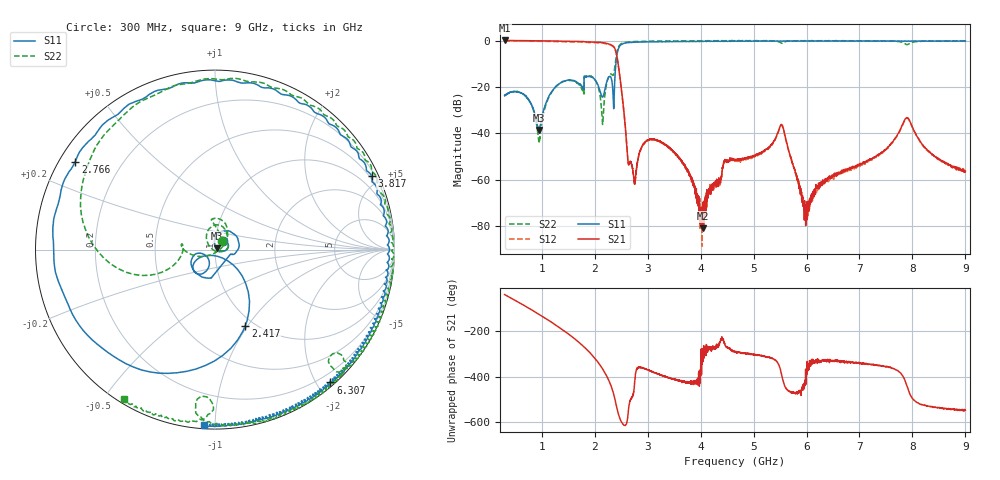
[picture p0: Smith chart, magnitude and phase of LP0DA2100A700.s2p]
!Agilent Technologies,E8358A,US41080443,A.07.50.56
!Agilent E8358A: A.07.50.56
!Date: Friday, August 05, 2016 08:45:06
!Correction: S11(Full 2 Port(1,2))
!S21(Full 2 Port(1,2))
!S12(Full 2 Port(1,2))
!S22(Full 2 Port(1,2))
!S2P File: Measurements: S11, S21, S12, S22:Log Frequency Sweep
# Hz S  dB  R 50
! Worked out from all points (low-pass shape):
!   6401 points, 300 MHz to 9 GHz, reference 50 ohm
!   highest |S21| = 0.06 dB at 301.1 MHz (marker M1); lowest = -81.0 dB at 4.043 GHz (marker M2)
!   |S21| within 3 dB of the highest: start of sweep to 2.371 GHz
!   lowest |S11| = -38.6 dB at 941.5 MHz (marker M3), VSWR 1.02, Z = 51 + j0.676 ohm
!   |S11| at or under -10 dB: start of sweep to 2.401 GHz
!   |S22| runs from -43.7 to 0.0 dB; largest |S21 - S12| = 0.028
!   S11 on the Smith chart (normalised r, x): 300 MHz: 1.09, +0.11; 2.417 GHz: 0.91, -0.98; 2.766 GHz: 0.05, +0.29; 3.817 GHz: 0.38, +4.44; 6.307 GHz: 0.06, -2.19; 9 GHz: 0.02, -0.94
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3e8  -23.71 47.7  0.06 -38.9  -0.17 -38.7  -23.78 50.7
3.011181e8  -23.71 47.7  0.06 -39.0  -0.18 -38.9  -23.74 50.5
7.380687e8  -24.97 -6.4  -0.03 -96.3  -0.25 -96.1  -25.12 -4.8
9.41463e8  -38.57 34.2  -0.05 -124.4  -0.28 -124.3  -42.71 -88.3
1.236527e9  -20.65 77.5  -0.17 -168.1  -0.40 -168.0  -20.78 121.5
1.75044e9  -19.54 -14.4  -0.39 101.6  -0.62 101.8  -20.48 43.3
1.985394e9  -16.36 -151.4  -0.65 46.8  -0.87 47.0  -16.18 67.7
2.137608e9  -24.21 -147.9  -0.84 -0.5  -1.07 -0.3  -32.54 -4.4
2.307614e9  -15.90 -139.8  -1.81 -78.4  -2.04 -78.3  -14.43 171.0
2.416812e9  -6.79 -68.4  -6.30 -173.8  -6.52 -173.8  -5.45 -167.5
2.632702e9  -0.92 178.7  -52.57 162.2  -52.62 161.5  -0.62 107.6
2.766089e9  -0.72 147.8  -60.06 -37.2  -60.10 -36.2  -0.38 84.9
3.201372e9  -0.54 81.2  -43.18 -28.0  -43.38 -28.0  -0.23 39.9
3.817078e9  -0.32 25.2  -58.84 -63.7  -59.23 -65.1  -0.05 3.4
4.042569e9  -0.39 11.3  -81.04 37.4  -77.62 7.1  -0.14 -5.6
4.651453e9  -0.21 -14.2  -51.54 69.1  -51.54 69.1  0.01 -24.3
5.525454e9  -0.22 -36.1  -36.23 -25.8  -36.49 -25.2  -1.12 -44.0
6.102778e9  -0.12 -45.7  -68.85 36.8  -69.21 15.2  -0.01 -52.7
6.307208e9  -0.17 -49.0  -60.12 34.1  -61.97 30.3  -0.06 -56.8
7.552286e9  -0.23 -69.5  -45.69 2.6  -45.83 2.8  -0.22 -87.1
7.918076e9  -0.17 -75.4  -33.44 -95.5  -33.69 -95.8  -1.59 -92.1
9e9  -0.21 -93.5  -56.42 174.1  -56.58 176.8  -0.20 -121.3
